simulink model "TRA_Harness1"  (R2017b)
settings: Solver=FixedStepDiscrete  StartTime=0.0  StopTime=16  FixedStep=0.01  RelTol=1e-3  EnableMultiTasking=on
undefined symbols (not defined in the file): sigbuilder_block
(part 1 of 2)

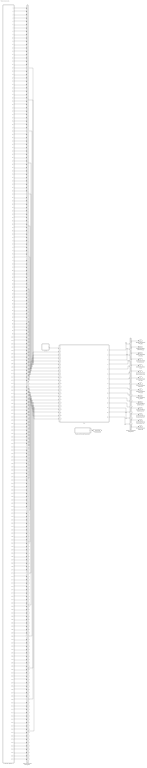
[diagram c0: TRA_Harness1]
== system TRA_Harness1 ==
  Chart : Stateflow chart  TreatAsAtomicUnit=on
  Harness Inputs : Subsystem  Tag=STV Subsys  LoadFcn=sigbuilder_block('load');  StartFcn=sigbuilder_block('start');  StopFcn=sigbuilder_block('stop');  ClipboardFcn=sigbuilder_block('clipboard');  mask(Sigbuilder block){tuvar=[0:10]}
      mask init:
      | if ~strcmp(get_param(bdroot(gcb),'SimulationStatus'),'stopped'),tuvar = sigbuilder_block('maskInit'); end
  Input Conversion Subsystem : Subsystem  Tag=__SLT_ICS__  Description=Signal spec. and routing
  Output Conversion Subsystem : Subsystem  Tag=__SLT_OCS__  Description=Signal spec. and routing
  Simulink Function scheduler : Test Sequence  Tag=__SLT_FCN_CALL__  TreatAsAtomicUnit=on
  TRA : ModelReference  ModelNameDialog=TRA  SimulationMode=Normal  ModelReferenceVersion='M112C123'
  GbTRA_ThmRnwyfDet_flg : Outport  OutDataTypeStr=boolean  PortDimensions=[1]
  GbTRA_TPLRnwyChkFinish_flg : Outport  Port=2  OutDataTypeStr=boolean  PortDimensions=[1]
  GbTRA_ShortSOCIDFit_flg : Outport  Port=3  OutDataTypeStr=boolean  PortDimensions=[1]
  GcTRA_ShortSOCMinID_numb : Outport  Port=4  OutDataTypeStr=uint8  PortDimensions=[1]
  GcTRA_RunTime_min : Outport  Port=5  OutDataTypeStr=uint16  PortDimensions=[1]
  GcTRA_ShortSOCRunTimeSum_min : Outport  Port=6  OutDataTypeStr=uint32  PortDimensions=[1]
  GcTRA_ShortSOCDiff_pct : Outport  Port=7  OutDataTypeStr=single  PortDimensions=[1]
  GbTRA_ThmRnwyWarn_flg : Outport  Port=8  OutDataTypeStr=boolean  PortDimensions=[1]
  GbTRA_ThmRnwyAlrm_flg : Outport  Port=9  OutDataTypeStr=boolean  PortDimensions=[1]
  GeTRA_ThmRnwySt_enum : Outport  Port=10  OutDataTypeStr=uint8  PortDimensions=[1]
  GcTRA_TPLWkupCellTemp_mV : Outport  Port=11  OutDataTypeStr=uint16  PortDimensions=[1]
  GcTRA_TPLWkupPCBTemp_mV : Outport  Port=12  OutDataTypeStr=uint16  PortDimensions=[1]
  GcTRA_TPLWkupCellVoltMax_mV : Outport  Port=13  OutDataTypeStr=uint16  PortDimensions=[1]
  GcTRA_TPLWkupCellVoltMin_mV : Outport  Port=14  OutDataTypeStr=uint16  PortDimensions=[1]
  GbTRA_TPLWkupEnable_flg : Outport  Port=15  OutDataTypeStr=boolean  PortDimensions=[1]
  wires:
  Harness Inputs/1(GcCDP_MaxCellTemp_C) -> Input Conversion Subsystem/1(Inport_1)
  Harness Inputs/2(GaCDP_CellTemp_C(1)) -> Input Conversion Subsystem/2(Inport_2)
  Harness Inputs/3(GaCDP_CellTemp_C(2)) -> Input Conversion Subsystem/3(Inport_3)
  Harness Inputs/4(GaCDP_CellTemp_C(3)) -> Input Conversion Subsystem/4(Inport_4)
  Harness Inputs/5(GaCDP_CellTemp_C(4)) -> Input Conversion Subsystem/5(Inport_5)
  Harness Inputs/6(GaCDP_CellTemp_C(5)) -> Input Conversion Subsystem/6(Inport_6)
  Harness Inputs/7(GaCDP_CellTemp_C(6)) -> Input Conversion Subsystem/7(Inport_7)
  Harness Inputs/8(GaCDP_CellTemp_C(7)) -> Input Conversion Subsystem/8(Inport_8)
  Harness Inputs/9(GaCDP_CellTemp_C(8)) -> Input Conversion Subsystem/9(Inport_9)
  Harness Inputs/10(GaCDP_CellTemp_C(9)) -> Input Conversion Subsystem/10(Inport_10)
  Harness Inputs/11(GaCDP_CellTemp_C(10)) -> Input Conversion Subsystem/11(Inport_11)
  Harness Inputs/12(GaCDP_CellTemp_C(11)) -> Input Conversion Subsystem/12(Inport_12)
  Harness Inputs/13(GaCDP_CellTemp_C(12)) -> Input Conversion Subsystem/13(Inport_13)
  Harness Inputs/14(GaCDP_CellTemp_C(13)) -> Input Conversion Subsystem/14(Inport_14)
  Harness Inputs/15(GaCDP_CellTemp_C(14)) -> Input Conversion Subsystem/15(Inport_15)
  Harness Inputs/16(GaCDP_CellTemp_C(15)) -> Input Conversion Subsystem/16(Inport_16)
  Harness Inputs/17(GaCDP_CellTemp_C(16)) -> Input Conversion Subsystem/17(Inport_17)
  Harness Inputs/18(GaCDP_CellTemp_C(17)) -> Input Conversion Subsystem/18(Inport_18)
  Harness Inputs/19(GaCDP_CellTemp_C(18)) -> Input Conversion Subsystem/19(Inport_19)
  Harness Inputs/20(GaCDP_CellTemp_C(19)) -> Input Conversion Subsystem/20(Inport_20)
  Harness Inputs/21(GaCDP_CellTemp_C(20)) -> Input Conversion Subsystem/21(Inport_21)
  Harness Inputs/22(GaCDP_CellTemp_C(21)) -> Input Conversion Subsystem/22(Inport_22)
  Harness Inputs/23(GaCDP_CellTemp_C(22)) -> Input Conversion Subsystem/23(Inport_23)
  Harness Inputs/24(GaCDP_CellTemp_C(23)) -> Input Conversion Subsystem/24(Inport_24)
  Harness Inputs/25(GaCDP_CellTemp_C(24)) -> Input Conversion Subsystem/25(Inport_25)
  Harness Inputs/26(GaCDP_CellTemp_C(25)) -> Input Conversion Subsystem/26(Inport_26)
  Harness Inputs/27(GaCDP_CellTemp_C(26)) -> Input Conversion Subsystem/27(Inport_27)
  Harness Inputs/28(GaCDP_CellTemp_C(27)) -> Input Conversion Subsystem/28(Inport_28)
  Harness Inputs/29(GaCDP_CellTemp_C(28)) -> Input Conversion Subsystem/29(Inport_29)
  Harness Inputs/30(GaCDP_CellTemp_C(29)) -> Input Conversion Subsystem/30(Inport_30)
  Harness Inputs/31(GaCDP_CellTemp_C(30)) -> Input Conversion Subsystem/31(Inport_31)
  Harness Inputs/32(GaCDP_CellTemp_C(31)) -> Input Conversion Subsystem/32(Inport_32)
  Harness Inputs/33(GaCDP_CellTemp_C(32)) -> Input Conversion Subsystem/33(Inport_33)
  Harness Inputs/34(GaCDP_CellTemp_C(33)) -> Input Conversion Subsystem/34(Inport_34)
  Harness Inputs/35(GaCDP_CellTemp_C(34)) -> Input Conversion Subsystem/35(Inport_35)
  Harness Inputs/36(GaCDP_CellTemp_C(35)) -> Input Conversion Subsystem/36(Inport_36)
  Harness Inputs/37(GaCDP_CellTemp_C(36)) -> Input Conversion Subsystem/37(Inport_37)
  Harness Inputs/38(GaCDP_CellTemp_C(37)) -> Input Conversion Subsystem/38(Inport_38)
  Harness Inputs/39(GaCDP_CellTemp_C(38)) -> Input Conversion Subsystem/39(Inport_39)
  Harness Inputs/40(GaCDP_CellTemp_C(39)) -> Input Conversion Subsystem/40(Inport_40)
  Harness Inputs/41(GaCDP_CellTemp_C(40)) -> Input Conversion Subsystem/41(Inport_41)
  Harness Inputs/42(GaCDP_CellTemp_C(41)) -> Input Conversion Subsystem/42(Inport_42)
  Harness Inputs/43(GaCDP_CellTemp_C(42)) -> Input Conversion Subsystem/43(Inport_43)
  Harness Inputs/44(GaCDP_CellTemp_C(43)) -> Input Conversion Subsystem/44(Inport_44)
  Harness Inputs/45(GaCDP_CellTemp_C(44)) -> Input Conversion Subsystem/45(Inport_45)
  Harness Inputs/46(GaCDP_CellTemp_C(45)) -> Input Conversion Subsystem/46(Inport_46)
  Harness Inputs/47(GaCDP_CellTemp_C(46)) -> Input Conversion Subsystem/47(Inport_47)
  Harness Inputs/48(GaCDP_CellTemp_C(47)) -> Input Conversion Subsystem/48(Inport_48)
  Harness Inputs/49(GaCDP_CellTemp_C(48)) -> Input Conversion Subsystem/49(Inport_49)
  Harness Inputs/50(GcCDP_MinCellTemp_C) -> Input Conversion Subsystem/50(Inport_50)
  Harness Inputs/51(GcUDS_CellTempNumb_numb) -> Input Conversion Subsystem/51(Inport_51)
  Harness Inputs/52(GcCDP_MaxBusbarTemp_C) -> Input Conversion Subsystem/52(Inport_52)
  Harness Inputs/53(GcCDP_MinBusbarTemp_C) -> Input Conversion Subsystem/53(Inport_53)
  Harness Inputs/54(GaCDP_BusbarTemp_C(1)) -> Input Conversion Subsystem/54(Inport_54)
  Harness Inputs/55(GaCDP_BusbarTemp_C(2)) -> Input Conversion Subsystem/55(Inport_55)
  Harness Inputs/56(GaCDP_BusbarTemp_C(3)) -> Input Conversion Subsystem/56(Inport_56)
  Harness Inputs/57(GaCDP_BusbarTemp_C(4)) -> Input Conversion Subsystem/57(Inport_57)
  Harness Inputs/58(GaCDP_BusbarTemp_C(5)) -> Input Conversion Subsystem/58(Inport_58)
  Harness Inputs/59(GaCDP_BusbarTemp_C(6)) -> Input Conversion Subsystem/59(Inport_59)
  Harness Inputs/60(GaCDP_BusbarTemp_C(7)) -> Input Conversion Subsystem/60(Inport_60)
  Harness Inputs/61(GaCDP_BusbarTemp_C(8)) -> Input Conversion Subsystem/61(Inport_61)
  Harness Inputs/62(GaCDP_BusbarTemp_C(9)) -> Input Conversion Subsystem/62(Inport_62)
  Harness Inputs/63(GaCDP_BusbarTemp_C(10)) -> Input Conversion Subsystem/63(Inport_63)
  Harness Inputs/64(GaCDP_BusbarTemp_C(11)) -> Input Conversion Subsystem/64(Inport_64)
  Harness Inputs/65(GaCDP_BusbarTemp_C(12)) -> Input Conversion Subsystem/65(Inport_65)
  Harness Inputs/66(GaCDP_BusbarTemp_C(13)) -> Input Conversion Subsystem/66(Inport_66)
  Harness Inputs/67(GaCDP_BusbarTemp_C(14)) -> Input Conversion Subsystem/67(Inport_67)
  Harness Inputs/68(GaCDP_BusbarTemp_C(15)) -> Input Conversion Subsystem/68(Inport_68)
  Harness Inputs/69(GaCDP_BusbarTemp_C(16)) -> Input Conversion Subsystem/69(Inport_69)
  Harness Inputs/70(GaCDP_BusbarTemp_C(17)) -> Input Conversion Subsystem/70(Inport_70)
  Harness Inputs/71(GaCDP_BusbarTemp_C(18)) -> Input Conversion Subsystem/71(Inport_71)
  Harness Inputs/72(GaCDP_BusbarTemp_C(19)) -> Input Conversion Subsystem/72(Inport_72)
  Harness Inputs/73(GaCDP_BusbarTemp_C(20)) -> Input Conversion Subsystem/73(Inport_73)
  Harness Inputs/74(GaCDP_BusbarTemp_C(21)) -> Input Conversion Subsystem/74(Inport_74)
  Harness Inputs/75(GaCDP_BusbarTemp_C(22)) -> Input Conversion Subsystem/75(Inport_75)
  Harness Inputs/76(GaCDP_BusbarTemp_C(23)) -> Input Conversion Subsystem/76(Inport_76)
  Harness Inputs/77(GaCDP_BusbarTemp_C(24)) -> Input Conversion Subsystem/77(Inport_77)
  Harness Inputs/78(GaCDP_BusbarTemp_C(25)) -> Input Conversion Subsystem/78(Inport_78)
  Harness Inputs/79(GaCDP_BusbarTemp_C(26)) -> Input Conversion Subsystem/79(Inport_79)
  Harness Inputs/80(GaCDP_BusbarTemp_C(27)) -> Input Conversion Subsystem/80(Inport_80)
  Harness Inputs/81(GaCDP_BusbarTemp_C(28)) -> Input Conversion Subsystem/81(Inport_81)
  Harness Inputs/82(GaCDP_BusbarTemp_C(29)) -> Input Conversion Subsystem/82(Inport_82)
  Harness Inputs/83(GaCDP_BusbarTemp_C(30)) -> Input Conversion Subsystem/83(Inport_83)
  Harness Inputs/84(GaCDP_BusbarTemp_C(31)) -> Input Conversion Subsystem/84(Inport_84)
  Harness Inputs/85(GaCDP_BusbarTemp_C(32)) -> Input Conversion Subsystem/85(Inport_85)
  Harness Inputs/86(GaCDP_BusbarTemp_C(33)) -> Input Conversion Subsystem/86(Inport_86)
  Harness Inputs/87(GaCDP_BusbarTemp_C(34)) -> Input Conversion Subsystem/87(Inport_87)
  Harness Inputs/88(GaCDP_BusbarTemp_C(35)) -> Input Conversion Subsystem/88(Inport_88)
  Harness Inputs/89(GaCDP_BusbarTemp_C(36)) -> Input Conversion Subsystem/89(Inport_89)
  Harness Inputs/90(GaCDP_BusbarTemp_C(37)) -> Input Conversion Subsystem/90(Inport_90)
  Harness Inputs/91(GaCDP_BusbarTemp_C(38)) -> Input Conversion Subsystem/91(Inport_91)
  Harness Inputs/92(GaCDP_BusbarTemp_C(39)) -> Input Conversion Subsystem/92(Inport_92)
  Harness Inputs/93(GaCDP_BusbarTemp_C(40)) -> Input Conversion Subsystem/93(Inport_93)
  Harness Inputs/94(GaCDP_BusbarTemp_C(41)) -> Input Conversion Subsystem/94(Inport_94)
  Harness Inputs/95(GaCDP_BusbarTemp_C(42)) -> Input Conversion Subsystem/95(Inport_95)
  Harness Inputs/96(GaCDP_BusbarTemp_C(43)) -> Input Conversion Subsystem/96(Inport_96)
  Harness Inputs/97(GaCDP_BusbarTemp_C(44)) -> Input Conversion Subsystem/97(Inport_97)
  Harness Inputs/98(GaCDP_BusbarTemp_C(45)) -> Input Conversion Subsystem/98(Inport_98)
  Harness Inputs/99(GaCDP_BusbarTemp_C(46)) -> Input Conversion Subsystem/99(Inport_99)
  Harness Inputs/100(GaCDP_BusbarTemp_C(47)) -> Input Conversion Subsystem/100(Inport_100)
  Harness Inputs/101(GaCDP_BusbarTemp_C(48)) -> Input Conversion Subsystem/101(Inport_101)
  Harness Inputs/102(GcUDS_BusbarTempNumb_numb) -> Input Conversion Subsystem/102(Inport_102)
  Harness Inputs/103(GeMSM_BMUState_enum) -> Input Conversion Subsystem/103(Inport_103)
  Harness Inputs/104(GbCDP_SumCellVoltVld_flg) -> Input Conversion Subsystem/104(Inport_104)
  Harness Inputs/105(GcRTC_SleepTime_min) -> Input Conversion Subsystem/105(Inport_105)
  Harness Inputs/106(GbNVM_ReadShortSOCIDFitVld_flg) -> Input Conversion Subsystem/106(Inport_106)
  Harness Inputs/107(GbNVM_ReadShortSOCMinIDVld_flg) -> Input Conversion Subsystem/107(Inport_107)
  Harness Inputs/108(GbNVM_ReadShortSOCDiffVld_flg) -> Input Conversion Subsystem/108(Inport_108)
  Harness Inputs/109(GbNVM_ReadShortSOCRunTiSumVld_flg) -> Input Conversion Subsystem/109(Inport_109)
  Harness Inputs/110(GaCDP_CellVolt_mV(1)) -> Input Conversion Subsystem/110(Inport_110)
  Harness Inputs/111(GaCDP_CellVolt_mV(2)) -> Input Conversion Subsystem/111(Inport_111)
  Harness Inputs/112(GaCDP_CellVolt_mV(3)) -> Input Conversion Subsystem/112(Inport_112)
  Harness Inputs/113(GaCDP_CellVolt_mV(4)) -> Input Conversion Subsystem/113(Inport_113)
  Harness Inputs/114(GaCDP_CellVolt_mV(5)) -> Input Conversion Subsystem/114(Inport_114)
  Harness Inputs/115(GaCDP_CellVolt_mV(6)) -> Input Conversion Subsystem/115(Inport_115)
  Harness Inputs/116(GaCDP_CellVolt_mV(7)) -> Input Conversion Subsystem/116(Inport_116)
  Harness Inputs/117(GaCDP_CellVolt_mV(8)) -> Input Conversion Subsystem/117(Inport_117)
  Harness Inputs/118(GaCDP_CellVolt_mV(9)) -> Input Conversion Subsystem/118(Inport_118)
  Harness Inputs/119(GaCDP_CellVolt_mV(10)) -> Input Conversion Subsystem/119(Inport_119)
  Harness Inputs/120(GaCDP_CellVolt_mV(11)) -> Input Conversion Subsystem/120(Inport_120)
  Harness Inputs/121(GaCDP_CellVolt_mV(12)) -> Input Conversion Subsystem/121(Inport_121)
  Harness Inputs/122(GaCDP_CellVolt_mV(13)) -> Input Conversion Subsystem/122(Inport_122)
  Harness Inputs/123(GaCDP_CellVolt_mV(14)) -> Input Conversion Subsystem/123(Inport_123)
  Harness Inputs/124(GaCDP_CellVolt_mV(15)) -> Input Conversion Subsystem/124(Inport_124)
  Harness Inputs/125(GaCDP_CellVolt_mV(16)) -> Input Conversion Subsystem/125(Inport_125)
  Harness Inputs/126(GaCDP_CellVolt_mV(17)) -> Input Conversion Subsystem/126(Inport_126)
  Harness Inputs/127(GaCDP_CellVolt_mV(18)) -> Input Conversion Subsystem/127(Inport_127)
  Harness Inputs/128(GaCDP_CellVolt_mV(19)) -> Input Conversion Subsystem/128(Inport_128)
  Harness Inputs/129(GaCDP_CellVolt_mV(20)) -> Input Conversion Subsystem/129(Inport_129)
  Harness Inputs/130(GaCDP_CellVolt_mV(21)) -> Input Conversion Subsystem/130(Inport_130)
  Harness Inputs/131(GaCDP_CellVolt_mV(22)) -> Input Conversion Subsystem/131(Inport_131)
  Harness Inputs/132(GaCDP_CellVolt_mV(23)) -> Input Conversion Subsystem/132(Inport_132)
  Harness Inputs/133(GaCDP_CellVolt_mV(24)) -> Input Conversion Subsystem/133(Inport_133)
  Harness Inputs/134(GaCDP_CellVolt_mV(25)) -> Input Conversion Subsystem/134(Inport_134)
  Harness Inputs/135(GaCDP_CellVolt_mV(26)) -> Input Conversion Subsystem/135(Inport_135)
  Harness Inputs/136(GaCDP_CellVolt_mV(27)) -> Input Conversion Subsystem/136(Inport_136)
  Harness Inputs/137(GaCDP_CellVolt_mV(28)) -> Input Conversion Subsystem/137(Inport_137)
  Harness Inputs/138(GaCDP_CellVolt_mV(29)) -> Input Conversion Subsystem/138(Inport_138)
  Harness Inputs/139(GaCDP_CellVolt_mV(30)) -> Input Conversion Subsystem/139(Inport_139)
  Harness Inputs/140(GaCDP_CellVolt_mV(31)) -> Input Conversion Subsystem/140(Inport_140)
  Harness Inputs/141(GaCDP_CellVolt_mV(32)) -> Input Conversion Subsystem/141(Inport_141)
  Harness Inputs/142(GaCDP_CellVolt_mV(33)) -> Input Conversion Subsystem/142(Inport_142)
  Harness Inputs/143(GaCDP_CellVolt_mV(34)) -> Input Conversion Subsystem/143(Inport_143)
  Harness Inputs/144(GaCDP_CellVolt_mV(35)) -> Input Conversion Subsystem/144(Inport_144)
  Harness Inputs/145(GaCDP_CellVolt_mV(36)) -> Input Conversion Subsystem/145(Inport_145)
  Harness Inputs/146(GaCDP_CellVolt_mV(37)) -> Input Conversion Subsystem/146(Inport_146)
  Harness Inputs/147(GaCDP_CellVolt_mV(38)) -> Input Conversion Subsystem/147(Inport_147)
  Harness Inputs/148(GaCDP_CellVolt_mV(39)) -> Input Conversion Subsystem/148(Inport_148)
  Harness Inputs/149(GaCDP_CellVolt_mV(40)) -> Input Conversion Subsystem/149(Inport_149)
  Harness Inputs/150(GaCDP_CellVolt_mV(41)) -> Input Conversion Subsystem/150(Inport_150)
  Harness Inputs/151(GaCDP_CellVolt_mV(42)) -> Input Conversion Subsystem/151(Inport_151)
  Harness Inputs/152(GaCDP_CellVolt_mV(43)) -> Input Conversion Subsystem/152(Inport_152)
  Harness Inputs/153(GaCDP_CellVolt_mV(44)) -> Input Conversion Subsystem/153(Inport_153)
  Harness Inputs/154(GaCDP_CellVolt_mV(45)) -> Input Conversion Subsystem/154(Inport_154)
  Harness Inputs/155(GaCDP_CellVolt_mV(46)) -> Input Conversion Subsystem/155(Inport_155)
  Harness Inputs/156(GaCDP_CellVolt_mV(47)) -> Input Conversion Subsystem/156(Inport_156)
  Harness Inputs/157(GaCDP_CellVolt_mV(48)) -> Input Conversion Subsystem/157(Inport_157)
  Harness Inputs/158(GaCDP_CellVolt_mV(49)) -> Input Conversion Subsystem/158(Inport_158)
  Harness Inputs/159(GaCDP_CellVolt_mV(50)) -> Input Conversion Subsystem/159(Inport_159)
  Harness Inputs/160(GaCDP_CellVolt_mV(51)) -> Input Conversion Subsystem/160(Inport_160)
  Harness Inputs/161(GaCDP_CellVolt_mV(52)) -> Input Conversion Subsystem/161(Inport_161)
  Harness Inputs/162(GaCDP_CellVolt_mV(53)) -> Input Conversion Subsystem/162(Inport_162)
  Harness Inputs/163(GaCDP_CellVolt_mV(54)) -> Input Conversion Subsystem/163(Inport_163)
  Harness Inputs/164(GaCDP_CellVolt_mV(55)) -> Input Conversion Subsystem/164(Inport_164)
  Harness Inputs/165(GaCDP_CellVolt_mV(56)) -> Input Conversion Subsystem/165(Inport_165)
  Harness Inputs/166(GaCDP_CellVolt_mV(57)) -> Input Conversion Subsystem/166(Inport_166)
  Harness Inputs/167(GaCDP_CellVolt_mV(58)) -> Input Conversion Subsystem/167(Inport_167)
  Harness Inputs/168(GaCDP_CellVolt_mV(59)) -> Input Conversion Subsystem/168(Inport_168)
  Harness Inputs/169(GaCDP_CellVolt_mV(60)) -> Input Conversion Subsystem/169(Inport_169)
  Harness Inputs/170(GaCDP_CellVolt_mV(61)) -> Input Conversion Subsystem/170(Inport_170)
  Harness Inputs/171(GaCDP_CellVolt_mV(62)) -> Input Conversion Subsystem/171(Inport_171)
  Harness Inputs/172(GaCDP_CellVolt_mV(63)) -> Input Conversion Subsystem/172(Inport_172)
  Harness Inputs/173(GaCDP_CellVolt_mV(64)) -> Input Conversion Subsystem/173(Inport_173)
  Harness Inputs/174(GaCDP_CellVolt_mV(65)) -> Input Conversion Subsystem/174(Inport_174)
  Harness Inputs/175(GaCDP_CellVolt_mV(66)) -> Input Conversion Subsystem/175(Inport_175)
  Harness Inputs/176(GaCDP_CellVolt_mV(67)) -> Input Conversion Subsystem/176(Inport_176)
  Harness Inputs/177(GaCDP_CellVolt_mV(68)) -> Input Conversion Subsystem/177(Inport_177)
  Harness Inputs/178(GaCDP_CellVolt_mV(69)) -> Input Conversion Subsystem/178(Inport_178)
  Harness Inputs/179(GaCDP_CellVolt_mV(70)) -> Input Conversion Subsystem/179(Inport_179)
  Harness Inputs/180(GaCDP_CellVolt_mV(71)) -> Input Conversion Subsystem/180(Inport_180)
  Harness Inputs/181(GaCDP_CellVolt_mV(72)) -> Input Conversion Subsystem/181(Inport_181)
  Harness Inputs/182(GaCDP_CellVolt_mV(73)) -> Input Conversion Subsystem/182(Inport_182)
  Harness Inputs/183(GaCDP_CellVolt_mV(74)) -> Input Conversion Subsystem/183(Inport_183)
  Harness Inputs/184(GaCDP_CellVolt_mV(75)) -> Input Conversion Subsystem/184(Inport_184)
  Harness Inputs/185(GaCDP_CellVolt_mV(76)) -> Input Conversion Subsystem/185(Inport_185)
  Harness Inputs/186(GaCDP_CellVolt_mV(77)) -> Input Conversion Subsystem/186(Inport_186)
  Harness Inputs/187(GaCDP_CellVolt_mV(78)) -> Input Conversion Subsystem/187(Inport_187)
  Harness Inputs/188(GaCDP_CellVolt_mV(79)) -> Input Conversion Subsystem/188(Inport_188)
  Harness Inputs/189(GaCDP_CellVolt_mV(80)) -> Input Conversion Subsystem/189(Inport_189)
  Harness Inputs/190(GaCDP_CellVolt_mV(81)) -> Input Conversion Subsystem/190(Inport_190)
  Harness Inputs/191(GaCDP_CellVolt_mV(82)) -> Input Conversion Subsystem/191(Inport_191)
  Harness Inputs/192(GaCDP_CellVolt_mV(83)) -> Input Conversion Subsystem/192(Inport_192)
  Harness Inputs/193(GaCDP_CellVolt_mV(84)) -> Input Conversion Subsystem/193(Inport_193)
  Harness Inputs/194(GaCDP_CellVolt_mV(85)) -> Input Conversion Subsystem/194(Inport_194)
  Harness Inputs/195(GaCDP_CellVolt_mV(86)) -> Input Conversion Subsystem/195(Inport_195)
  Harness Inputs/196(GaCDP_CellVolt_mV(87)) -> Input Conversion Subsystem/196(Inport_196)
  Harness Inputs/197(GaCDP_CellVolt_mV(88)) -> Input Conversion Subsystem/197(Inport_197)
  Harness Inputs/198(GaCDP_CellVolt_mV(89)) -> Input Conversion Subsystem/198(Inport_198)
  Harness Inputs/199(GaCDP_CellVolt_mV(90)) -> Input Conversion Subsystem/199(Inport_199)
  Harness Inputs/200(GaCDP_CellVolt_mV(91)) -> Input Conversion Subsystem/200(Inport_200)
  Harness Inputs/201(GaCDP_CellVolt_mV(92)) -> Input Conversion Subsystem/201(Inport_201)
  Harness Inputs/202(GaCDP_CellVolt_mV(93)) -> Input Conversion Subsystem/202(Inport_202)
  Harness Inputs/203(GaCDP_CellVolt_mV(94)) -> Input Conversion Subsystem/203(Inport_203)
  Harness Inputs/204(GaCDP_CellVolt_mV(95)) -> Input Conversion Subsystem/204(Inport_204)
  Harness Inputs/205(GaCDP_CellVolt_mV(96)) -> Input Conversion Subsystem/205(Inport_205)
  Harness Inputs/206(GaCDP_CellVolt_mV(97)) -> Input Conversion Subsystem/206(Inport_206)
  Harness Inputs/207(GaCDP_CellVolt_mV(98)) -> Input Conversion Subsystem/207(Inport_207)
  Harness Inputs/208(GaCDP_CellVolt_mV(99)) -> Input Conversion Subsystem/208(Inport_208)
  Harness Inputs/209(GaCDP_CellVolt_mV(100)) -> Input Conversion Subsystem/209(Inport_209)
  Harness Inputs/210(GaCDP_CellVolt_mV(101)) -> Input Conversion Subsystem/210(Inport_210)
  Harness Inputs/211(GaCDP_CellVolt_mV(102)) -> Input Conversion Subsystem/211(Inport_211)
  Harness Inputs/212(GaCDP_CellVolt_mV(103)) -> Input Conversion Subsystem/212(Inport_212)
  Harness Inputs/213(GaCDP_CellVolt_mV(104)) -> Input Conversion Subsystem/213(Inport_213)
  Harness Inputs/214(GaCDP_CellVolt_mV(105)) -> Input Conversion Subsystem/214(Inport_214)
  Harness Inputs/215(GaCDP_CellVolt_mV(106)) -> Input Conversion Subsystem/215(Inport_215)
  Harness Inputs/216(GaCDP_CellVolt_mV(107)) -> Input Conversion Subsystem/216(Inport_216)
  Harness Inputs/217(GaCDP_CellVolt_mV(108)) -> Input Conversion Subsystem/217(Inport_217)
  Harness Inputs/218(GaCDP_CellVolt_mV(109)) -> Input Conversion Subsystem/218(Inport_218)
  Harness Inputs/219(GaCDP_CellVolt_mV(110)) -> Input Conversion Subsystem/219(Inport_219)
  Harness Inputs/220(GaCDP_CellVolt_mV(111)) -> Input Conversion Subsystem/220(Inport_220)
  Harness Inputs/221(GaCDP_CellVolt_mV(112)) -> Input Conversion Subsystem/221(Inport_221)
  Harness Inputs/222(GeUDS_CapSel_enum) -> Input Conversion Subsystem/222(Inport_222)
  Harness Inputs/223(GbNVM_ReadLastShortSOCRunTiVld_flg) -> Input Conversion Subsystem/223(Inport_223)
  Harness Inputs/224(GcCDP_AvgCellVolt_mV) -> Input Conversion Subsystem/224(Inport_224)
  Harness Inputs/225(GcUDS_CellVoltNum_numb) -> Input Conversion Subsystem/225(Inport_225)
  Harness Inputs/226(GcHDP_PackCrnt_A) -> Input Conversion Subsystem/226(Inport_226)
  Harness Inputs/227(GeISP_WkUpSrcSt_enum) -> Input Conversion Subsystem/227(Inport_227)
  Output Conversion Subsystem/1(Outport_1) -> GbTRA_ThmRnwyfDet_flg/1
  Output Conversion Subsystem/2(Outport_2) -> GbTRA_TPLRnwyChkFinish_flg/1
  Output Conversion Subsystem/3(Outport_3) -> GbTRA_ShortSOCIDFit_flg/1
  Output Conversion Subsystem/4(Outport_4) -> GcTRA_ShortSOCMinID_numb/1
  Output Conversion Subsystem/5(Outport_5) -> GcTRA_RunTime_min/1
  Output Conversion Subsystem/6(Outport_6) -> GcTRA_ShortSOCRunTimeSum_min/1
  Output Conversion Subsystem/7(Outport_7) -> GcTRA_ShortSOCDiff_pct/1
  Output Conversion Subsystem/8(Outport_8) -> GbTRA_ThmRnwyWarn_flg/1
  Output Conversion Subsystem/9(Outport_9) -> GbTRA_ThmRnwyAlrm_flg/1
  Output Conversion Subsystem/10(Outport_10) -> GeTRA_ThmRnwySt_enum/1
  Output Conversion Subsystem/11(Outport_11) -> GcTRA_TPLWkupCellTemp_mV/1
  Output Conversion Subsystem/12(Outport_12) -> GcTRA_TPLWkupPCBTemp_mV/1
  Output Conversion Subsystem/13(Outport_13) -> GcTRA_TPLWkupCellVoltMax_mV/1
  Output Conversion Subsystem/14(Outport_14) -> GcTRA_TPLWkupCellVoltMin_mV/1
  Output Conversion Subsystem/15(Outport_15) -> GbTRA_TPLWkupEnable_flg/1
  Input Conversion Subsystem/2(Outport_2) -> TRA/2
  Input Conversion Subsystem/3(Outport_3) -> TRA/3
  Input Conversion Subsystem/4(Outport_4) -> TRA/4
  Input Conversion Subsystem/5(Outport_5) -> TRA/5
  Input Conversion Subsystem/6(Outport_6) -> TRA/6
  Input Conversion Subsystem/7(Outport_7) -> TRA/7
  Input Conversion Subsystem/8(Outport_8) -> TRA/8
  Input Conversion Subsystem/9(Outport_9) -> TRA/9
  Input Conversion Subsystem/10(Outport_10) -> TRA/10
  Input Conversion Subsystem/11(Outport_11) -> TRA/11
  Input Conversion Subsystem/12(Outport_12) -> TRA/12
  Input Conversion Subsystem/13(Outport_13) -> TRA/13
  Input Conversion Subsystem/14(Outport_14) -> TRA/14
  Input Conversion Subsystem/15(Outport_15) -> TRA/15
  Input Conversion Subsystem/16(Outport_16) -> TRA/16
  Input Conversion Subsystem/17(Outport_17) -> TRA/17
  Input Conversion Subsystem/18(Outport_18) -> TRA/18
  Input Conversion Subsystem/19(Outport_19) -> TRA/19
  Input Conversion Subsystem/20(Outport_20) -> TRA/20
  Input Conversion Subsystem/21(Outport_21) -> TRA/21
  Input Conversion Subsystem/22(Outport_22) -> TRA/22
  Input Conversion Subsystem/23(Outport_23) -> TRA/23
  TRA/1 -> Output Conversion Subsystem/1(Inport_1)
  TRA/2 -> Output Conversion Subsystem/2(Inport_2)
  TRA/3 -> Output Conversion Subsystem/3(Inport_3)
  TRA/4 -> Output Conversion Subsystem/4(Inport_4)
  TRA/5 -> Output Conversion Subsystem/5(Inport_5)
  TRA/6 -> Output Conversion Subsystem/6(Inport_6)
  TRA/7 -> Output Conversion Subsystem/7(Inport_7)
  TRA/8 -> Output Conversion Subsystem/8(Inport_8)
  TRA/9 -> Output Conversion Subsystem/9(Inport_9)
  TRA/10 -> Output Conversion Subsystem/10(Inport_10)
  TRA/11 -> Output Conversion Subsystem/11(Inport_11)
  TRA/12 -> Output Conversion Subsystem/12(Inport_12)
  TRA/13 -> Output Conversion Subsystem/13(Inport_13)
  TRA/14 -> Output Conversion Subsystem/14(Inport_14)
  TRA/15 -> Output Conversion Subsystem/15(Inport_15)
  Simulink Function scheduler/1(TRA_ThemRunAway_10ms()) -> [send_fcn1]
  Chart/1(Run10ms()) -> TRA/1

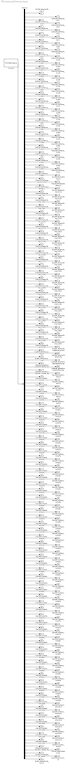
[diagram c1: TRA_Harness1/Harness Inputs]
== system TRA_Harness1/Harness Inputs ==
  Demux : Demux  Tag=STV Demux  Outputs=227
  FromWs : FromWorkspace  Tag=STV FromWs  VariableName=tuvar  SampleTime=0
  GcCDP_MaxCellTemp_C : Outport  Tag=STV Outport
  GaCDP_CellTemp_C(1) : Outport  Tag=STV Outport  Port=2
  GaCDP_CellTemp_C(2) : Outport  Tag=STV Outport  Port=3
  GaCDP_CellTemp_C(3) : Outport  Tag=STV Outport  Port=4
  GaCDP_CellTemp_C(4) : Outport  Tag=STV Outport  Port=5
  GaCDP_CellTemp_C(5) : Outport  Tag=STV Outport  Port=6
  GaCDP_CellTemp_C(6) : Outport  Tag=STV Outport  Port=7
  GaCDP_CellTemp_C(7) : Outport  Tag=STV Outport  Port=8
  GaCDP_CellTemp_C(8) : Outport  Tag=STV Outport  Port=9
  GaCDP_CellTemp_C(9) : Outport  Tag=STV Outport  Port=10
  GaCDP_CellTemp_C(10) : Outport  Tag=STV Outport  Port=11
  GaCDP_CellTemp_C(11) : Outport  Tag=STV Outport  Port=12
  GaCDP_CellTemp_C(12) : Outport  Tag=STV Outport  Port=13
  GaCDP_CellTemp_C(13) : Outport  Tag=STV Outport  Port=14
  GaCDP_CellTemp_C(14) : Outport  Tag=STV Outport  Port=15
  GaCDP_CellTemp_C(15) : Outport  Tag=STV Outport  Port=16
  GaCDP_CellTemp_C(16) : Outport  Tag=STV Outport  Port=17
  GaCDP_CellTemp_C(17) : Outport  Tag=STV Outport  Port=18
  GaCDP_CellTemp_C(18) : Outport  Tag=STV Outport  Port=19
  GaCDP_CellTemp_C(19) : Outport  Tag=STV Outport  Port=20
  GaCDP_CellTemp_C(20) : Outport  Tag=STV Outport  Port=21
  GaCDP_CellTemp_C(21) : Outport  Tag=STV Outport  Port=22
  GaCDP_CellTemp_C(22) : Outport  Tag=STV Outport  Port=23
  GaCDP_CellTemp_C(23) : Outport  Tag=STV Outport  Port=24
  GaCDP_CellTemp_C(24) : Outport  Tag=STV Outport  Port=25
  GaCDP_CellTemp_C(25) : Outport  Tag=STV Outport  Port=26
  GaCDP_CellTemp_C(26) : Outport  Tag=STV Outport  Port=27
  GaCDP_CellTemp_C(27) : Outport  Tag=STV Outport  Port=28
  GaCDP_CellTemp_C(28) : Outport  Tag=STV Outport  Port=29
  GaCDP_CellTemp_C(29) : Outport  Tag=STV Outport  Port=30
  GaCDP_CellTemp_C(30) : Outport  Tag=STV Outport  Port=31
  GaCDP_CellTemp_C(31) : Outport  Tag=STV Outport  Port=32
  GaCDP_CellTemp_C(32) : Outport  Tag=STV Outport  Port=33
  GaCDP_CellTemp_C(33) : Outport  Tag=STV Outport  Port=34
  GaCDP_CellTemp_C(34) : Outport  Tag=STV Outport  Port=35
  GaCDP_CellTemp_C(35) : Outport  Tag=STV Outport  Port=36
  GaCDP_CellTemp_C(36) : Outport  Tag=STV Outport  Port=37
  GaCDP_CellTemp_C(37) : Outport  Tag=STV Outport  Port=38
  GaCDP_CellTemp_C(38) : Outport  Tag=STV Outport  Port=39
  GaCDP_CellTemp_C(39) : Outport  Tag=STV Outport  Port=40
  GaCDP_CellTemp_C(40) : Outport  Tag=STV Outport  Port=41
  GaCDP_CellTemp_C(41) : Outport  Tag=STV Outport  Port=42
  GaCDP_CellTemp_C(42) : Outport  Tag=STV Outport  Port=43
  GaCDP_CellTemp_C(43) : Outport  Tag=STV Outport  Port=44
  GaCDP_CellTemp_C(44) : Outport  Tag=STV Outport  Port=45
  GaCDP_CellTemp_C(45) : Outport  Tag=STV Outport  Port=46
  GaCDP_CellTemp_C(46) : Outport  Tag=STV Outport  Port=47
  GaCDP_CellTemp_C(47) : Outport  Tag=STV Outport  Port=48
  GaCDP_CellTemp_C(48) : Outport  Tag=STV Outport  Port=49
  GcCDP_MinCellTemp_C : Outport  Tag=STV Outport  Port=50
  GcUDS_CellTempNumb_numb : Outport  Tag=STV Outport  Port=51
  GcCDP_MaxBusbarTemp_C : Outport  Tag=STV Outport  Port=52
  GcCDP_MinBusbarTemp_C : Outport  Tag=STV Outport  Port=53
  GaCDP_BusbarTemp_C(1) : Outport  Tag=STV Outport  Port=54
  GaCDP_BusbarTemp_C(2) : Outport  Tag=STV Outport  Port=55
  GaCDP_BusbarTemp_C(3) : Outport  Tag=STV Outport  Port=56
  GaCDP_BusbarTemp_C(4) : Outport  Tag=STV Outport  Port=57
  GaCDP_BusbarTemp_C(5) : Outport  Tag=STV Outport  Port=58
  GaCDP_BusbarTemp_C(6) : Outport  Tag=STV Outport  Port=59
  GaCDP_BusbarTemp_C(7) : Outport  Tag=STV Outport  Port=60
  GaCDP_BusbarTemp_C(8) : Outport  Tag=STV Outport  Port=61
  GaCDP_BusbarTemp_C(9) : Outport  Tag=STV Outport  Port=62
  GaCDP_BusbarTemp_C(10) : Outport  Tag=STV Outport  Port=63
  GaCDP_BusbarTemp_C(11) : Outport  Tag=STV Outport  Port=64
  GaCDP_BusbarTemp_C(12) : Outport  Tag=STV Outport  Port=65
  GaCDP_BusbarTemp_C(13) : Outport  Tag=STV Outport  Port=66
  GaCDP_BusbarTemp_C(14) : Outport  Tag=STV Outport  Port=67
  GaCDP_BusbarTemp_C(15) : Outport  Tag=STV Outport  Port=68
  GaCDP_BusbarTemp_C(16) : Outport  Tag=STV Outport  Port=69
  GaCDP_BusbarTemp_C(17) : Outport  Tag=STV Outport  Port=70
  GaCDP_BusbarTemp_C(18) : Outport  Tag=STV Outport  Port=71
  GaCDP_BusbarTemp_C(19) : Outport  Tag=STV Outport  Port=72
  GaCDP_BusbarTemp_C(20) : Outport  Tag=STV Outport  Port=73
  GaCDP_BusbarTemp_C(21) : Outport  Tag=STV Outport  Port=74
  GaCDP_BusbarTemp_C(22) : Outport  Tag=STV Outport  Port=75
  GaCDP_BusbarTemp_C(23) : Outport  Tag=STV Outport  Port=76
  GaCDP_BusbarTemp_C(24) : Outport  Tag=STV Outport  Port=77
  GaCDP_BusbarTemp_C(25) : Outport  Tag=STV Outport  Port=78
  GaCDP_BusbarTemp_C(26) : Outport  Tag=STV Outport  Port=79
  GaCDP_BusbarTemp_C(27) : Outport  Tag=STV Outport  Port=80
  GaCDP_BusbarTemp_C(28) : Outport  Tag=STV Outport  Port=81
  GaCDP_BusbarTemp_C(29) : Outport  Tag=STV Outport  Port=82
  GaCDP_BusbarTemp_C(30) : Outport  Tag=STV Outport  Port=83
  GaCDP_BusbarTemp_C(31) : Outport  Tag=STV Outport  Port=84
  GaCDP_BusbarTemp_C(32) : Outport  Tag=STV Outport  Port=85
  GaCDP_BusbarTemp_C(33) : Outport  Tag=STV Outport  Port=86
  GaCDP_BusbarTemp_C(34) : Outport  Tag=STV Outport  Port=87
  GaCDP_BusbarTemp_C(35) : Outport  Tag=STV Outport  Port=88
  GaCDP_BusbarTemp_C(36) : Outport  Tag=STV Outport  Port=89
  GaCDP_BusbarTemp_C(37) : Outport  Tag=STV Outport  Port=90
  GaCDP_BusbarTemp_C(38) : Outport  Tag=STV Outport  Port=91
  GaCDP_BusbarTemp_C(39) : Outport  Tag=STV Outport  Port=92
  GaCDP_BusbarTemp_C(40) : Outport  Tag=STV Outport  Port=93
  GaCDP_BusbarTemp_C(41) : Outport  Tag=STV Outport  Port=94
  GaCDP_BusbarTemp_C(42) : Outport  Tag=STV Outport  Port=95
  GaCDP_BusbarTemp_C(43) : Outport  Tag=STV Outport  Port=96
  GaCDP_BusbarTemp_C(44) : Outport  Tag=STV Outport  Port=97
  GaCDP_BusbarTemp_C(45) : Outport  Tag=STV Outport  Port=98
  GaCDP_BusbarTemp_C(46) : Outport  Tag=STV Outport  Port=99
  GaCDP_BusbarTemp_C(47) : Outport  Tag=STV Outport  Port=100
  GaCDP_BusbarTemp_C(48) : Outport  Tag=STV Outport  Port=101
  GcUDS_BusbarTempNumb_numb : Outport  Tag=STV Outport  Port=102
  GeMSM_BMUState_enum : Outport  Tag=STV Outport  Port=103
  GbCDP_SumCellVoltVld_flg : Outport  Tag=STV Outport  Port=104
  GcRTC_SleepTime_min : Outport  Tag=STV Outport  Port=105
  GbNVM_ReadShortSOCIDFitVld_flg : Outport  Tag=STV Outport  Port=106
  GbNVM_ReadShortSOCMinIDVld_flg : Outport  Tag=STV Outport  Port=107
  GbNVM_ReadShortSOCDiffVld_flg : Outport  Tag=STV Outport  Port=108
  GbNVM_ReadShortSOCRunTiSumVld_flg : Outport  Tag=STV Outport  Port=109
  GaCDP_CellVolt_mV(1) : Outport  Tag=STV Outport  Port=110
  GaCDP_CellVolt_mV(2) : Outport  Tag=STV Outport  Port=111
  GaCDP_CellVolt_mV(3) : Outport  Tag=STV Outport  Port=112
  GaCDP_CellVolt_mV(4) : Outport  Tag=STV Outport  Port=113
  GaCDP_CellVolt_mV(5) : Outport  Tag=STV Outport  Port=114
  GaCDP_CellVolt_mV(6) : Outport  Tag=STV Outport  Port=115
  GaCDP_CellVolt_mV(7) : Outport  Tag=STV Outport  Port=116
  GaCDP_CellVolt_mV(8) : Outport  Tag=STV Outport  Port=117
  GaCDP_CellVolt_mV(9) : Outport  Tag=STV Outport  Port=118
  GaCDP_CellVolt_mV(10) : Outport  Tag=STV Outport  Port=119
  GaCDP_CellVolt_mV(11) : Outport  Tag=STV Outport  Port=120
  GaCDP_CellVolt_mV(12) : Outport  Tag=STV Outport  Port=121
  GaCDP_CellVolt_mV(13) : Outport  Tag=STV Outport  Port=122
  GaCDP_CellVolt_mV(14) : Outport  Tag=STV Outport  Port=123
  GaCDP_CellVolt_mV(15) : Outport  Tag=STV Outport  Port=124
  GaCDP_CellVolt_mV(16) : Outport  Tag=STV Outport  Port=125
  GaCDP_CellVolt_mV(17) : Outport  Tag=STV Outport  Port=126
  GaCDP_CellVolt_mV(18) : Outport  Tag=STV Outport  Port=127
  GaCDP_CellVolt_mV(19) : Outport  Tag=STV Outport  Port=128
  GaCDP_CellVolt_mV(20) : Outport  Tag=STV Outport  Port=129
  GaCDP_CellVolt_mV(21) : Outport  Tag=STV Outport  Port=130
  GaCDP_CellVolt_mV(22) : Outport  Tag=STV Outport  Port=131
  GaCDP_CellVolt_mV(23) : Outport  Tag=STV Outport  Port=132
  GaCDP_CellVolt_mV(24) : Outport  Tag=STV Outport  Port=133
  GaCDP_CellVolt_mV(25) : Outport  Tag=STV Outport  Port=134
  GaCDP_CellVolt_mV(26) : Outport  Tag=STV Outport  Port=135
  GaCDP_CellVolt_mV(27) : Outport  Tag=STV Outport  Port=136
  GaCDP_CellVolt_mV(28) : Outport  Tag=STV Outport  Port=137
  GaCDP_CellVolt_mV(29) : Outport  Tag=STV Outport  Port=138
  GaCDP_CellVolt_mV(30) : Outport  Tag=STV Outport  Port=139
  GaCDP_CellVolt_mV(31) : Outport  Tag=STV Outport  Port=140
  GaCDP_CellVolt_mV(32) : Outport  Tag=STV Outport  Port=141
  GaCDP_CellVolt_mV(33) : Outport  Tag=STV Outport  Port=142
  GaCDP_CellVolt_mV(34) : Outport  Tag=STV Outport  Port=143
  GaCDP_CellVolt_mV(35) : Outport  Tag=STV Outport  Port=144
  GaCDP_CellVolt_mV(36) : Outport  Tag=STV Outport  Port=145
  GaCDP_CellVolt_mV(37) : Outport  Tag=STV Outport  Port=146
  GaCDP_CellVolt_mV(38) : Outport  Tag=STV Outport  Port=147
  GaCDP_CellVolt_mV(39) : Outport  Tag=STV Outport  Port=148
  GaCDP_CellVolt_mV(40) : Outport  Tag=STV Outport  Port=149
  GaCDP_CellVolt_mV(41) : Outport  Tag=STV Outport  Port=150
  GaCDP_CellVolt_mV(42) : Outport  Tag=STV Outport  Port=151
  GaCDP_CellVolt_mV(43) : Outport  Tag=STV Outport  Port=152
  GaCDP_CellVolt_mV(44) : Outport  Tag=STV Outport  Port=153
  GaCDP_CellVolt_mV(45) : Outport  Tag=STV Outport  Port=154
  GaCDP_CellVolt_mV(46) : Outport  Tag=STV Outport  Port=155
  GaCDP_CellVolt_mV(47) : Outport  Tag=STV Outport  Port=156
  GaCDP_CellVolt_mV(48) : Outport  Tag=STV Outport  Port=157
  GaCDP_CellVolt_mV(49) : Outport  Tag=STV Outport  Port=158
  GaCDP_CellVolt_mV(50) : Outport  Tag=STV Outport  Port=159
  GaCDP_CellVolt_mV(51) : Outport  Tag=STV Outport  Port=160
  GaCDP_CellVolt_mV(52) : Outport  Tag=STV Outport  Port=161
  GaCDP_CellVolt_mV(53) : Outport  Tag=STV Outport  Port=162
  GaCDP_CellVolt_mV(54) : Outport  Tag=STV Outport  Port=163
  GaCDP_CellVolt_mV(55) : Outport  Tag=STV Outport  Port=164
  GaCDP_CellVolt_mV(56) : Outport  Tag=STV Outport  Port=165
  GaCDP_CellVolt_mV(57) : Outport  Tag=STV Outport  Port=166
  GaCDP_CellVolt_mV(58) : Outport  Tag=STV Outport  Port=167
  GaCDP_CellVolt_mV(59) : Outport  Tag=STV Outport  Port=168
  GaCDP_CellVolt_mV(60) : Outport  Tag=STV Outport  Port=169
  GaCDP_CellVolt_mV(61) : Outport  Tag=STV Outport  Port=170
  GaCDP_CellVolt_mV(62) : Outport  Tag=STV Outport  Port=171
  GaCDP_CellVolt_mV(63) : Outport  Tag=STV Outport  Port=172
  GaCDP_CellVolt_mV(64) : Outport  Tag=STV Outport  Port=173
  GaCDP_CellVolt_mV(65) : Outport  Tag=STV Outport  Port=174
  GaCDP_CellVolt_mV(66) : Outport  Tag=STV Outport  Port=175
  GaCDP_CellVolt_mV(67) : Outport  Tag=STV Outport  Port=176
  GaCDP_CellVolt_mV(68) : Outport  Tag=STV Outport  Port=177
  GaCDP_CellVolt_mV(69) : Outport  Tag=STV Outport  Port=178
  GaCDP_CellVolt_mV(70) : Outport  Tag=STV Outport  Port=179
  GaCDP_CellVolt_mV(71) : Outport  Tag=STV Outport  Port=180
  GaCDP_CellVolt_mV(72) : Outport  Tag=STV Outport  Port=181
  GaCDP_CellVolt_mV(73) : Outport  Tag=STV Outport  Port=182
  GaCDP_CellVolt_mV(74) : Outport  Tag=STV Outport  Port=183
  GaCDP_CellVolt_mV(75) : Outport  Tag=STV Outport  Port=184
  GaCDP_CellVolt_mV(76) : Outport  Tag=STV Outport  Port=185
  GaCDP_CellVolt_mV(77) : Outport  Tag=STV Outport  Port=186
  GaCDP_CellVolt_mV(78) : Outport  Tag=STV Outport  Port=187
  GaCDP_CellVolt_mV(79) : Outport  Tag=STV Outport  Port=188
  GaCDP_CellVolt_mV(80) : Outport  Tag=STV Outport  Port=189
  GaCDP_CellVolt_mV(81) : Outport  Tag=STV Outport  Port=190
  GaCDP_CellVolt_mV(82) : Outport  Tag=STV Outport  Port=191
  GaCDP_CellVolt_mV(83) : Outport  Tag=STV Outport  Port=192
  GaCDP_CellVolt_mV(84) : Outport  Tag=STV Outport  Port=193
  GaCDP_CellVolt_mV(85) : Outport  Tag=STV Outport  Port=194
  GaCDP_CellVolt_mV(86) : Outport  Tag=STV Outport  Port=195
  GaCDP_CellVolt_mV(87) : Outport  Tag=STV Outport  Port=196
  GaCDP_CellVolt_mV(88) : Outport  Tag=STV Outport  Port=197
  GaCDP_CellVolt_mV(89) : Outport  Tag=STV Outport  Port=198
  GaCDP_CellVolt_mV(90) : Outport  Tag=STV Outport  Port=199
  GaCDP_CellVolt_mV(91) : Outport  Tag=STV Outport  Port=200
  GaCDP_CellVolt_mV(92) : Outport  Tag=STV Outport  Port=201
  GaCDP_CellVolt_mV(93) : Outport  Tag=STV Outport  Port=202
  GaCDP_CellVolt_mV(94) : Outport  Tag=STV Outport  Port=203
  GaCDP_CellVolt_mV(95) : Outport  Tag=STV Outport  Port=204
  GaCDP_CellVolt_mV(96) : Outport  Tag=STV Outport  Port=205
  GaCDP_CellVolt_mV(97) : Outport  Tag=STV Outport  Port=206
  GaCDP_CellVolt_mV(98) : Outport  Tag=STV Outport  Port=207
  GaCDP_CellVolt_mV(99) : Outport  Tag=STV Outport  Port=208
  GaCDP_CellVolt_mV(100) : Outport  Tag=STV Outport  Port=209
  GaCDP_CellVolt_mV(101) : Outport  Tag=STV Outport  Port=210
  GaCDP_CellVolt_mV(102) : Outport  Tag=STV Outport  Port=211
  GaCDP_CellVolt_mV(103) : Outport  Tag=STV Outport  Port=212
  GaCDP_CellVolt_mV(104) : Outport  Tag=STV Outport  Port=213
  GaCDP_CellVolt_mV(105) : Outport  Tag=STV Outport  Port=214
  GaCDP_CellVolt_mV(106) : Outport  Tag=STV Outport  Port=215
  GaCDP_CellVolt_mV(107) : Outport  Tag=STV Outport  Port=216
  GaCDP_CellVolt_mV(108) : Outport  Tag=STV Outport  Port=217
  GaCDP_CellVolt_mV(109) : Outport  Tag=STV Outport  Port=218
  GaCDP_CellVolt_mV(110) : Outport  Tag=STV Outport  Port=219
  GaCDP_CellVolt_mV(111) : Outport  Tag=STV Outport  Port=220
  GaCDP_CellVolt_mV(112) : Outport  Tag=STV Outport  Port=221
  GeUDS_CapSel_enum : Outport  Tag=STV Outport  Port=222
  GbNVM_ReadLastShortSOCRunTiVld_flg : Outport  Tag=STV Outport  Port=223
  GcCDP_AvgCellVolt_mV : Outport  Tag=STV Outport  Port=224
  GcUDS_CellVoltNum_numb : Outport  Tag=STV Outport  Port=225
  GcHDP_PackCrnt_A : Outport  Tag=STV Outport  Port=226
  GeISP_WkUpSrcSt_enum : Outport  Tag=STV Outport  Port=227
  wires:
  FromWs/1 -> Demux/1
  Demux/1 -> GcCDP_MaxCellTemp_C/1
  Demux/2 -> GaCDP_CellTemp_C(1)/1
  Demux/3 -> GaCDP_CellTemp_C(2)/1
  Demux/4 -> GaCDP_CellTemp_C(3)/1
  Demux/5 -> GaCDP_CellTemp_C(4)/1
  Demux/6 -> GaCDP_CellTemp_C(5)/1
  Demux/7 -> GaCDP_CellTemp_C(6)/1
  Demux/8 -> GaCDP_CellTemp_C(7)/1
  Demux/9 -> GaCDP_CellTemp_C(8)/1
  Demux/10 -> GaCDP_CellTemp_C(9)/1
  Demux/11 -> GaCDP_CellTemp_C(10)/1
  Demux/12 -> GaCDP_CellTemp_C(11)/1
  Demux/13 -> GaCDP_CellTemp_C(12)/1
  Demux/14 -> GaCDP_CellTemp_C(13)/1
  Demux/15 -> GaCDP_CellTemp_C(14)/1
  Demux/16 -> GaCDP_CellTemp_C(15)/1
  Demux/17 -> GaCDP_CellTemp_C(16)/1
  Demux/18 -> GaCDP_CellTemp_C(17)/1
  Demux/19 -> GaCDP_CellTemp_C(18)/1
  Demux/20 -> GaCDP_CellTemp_C(19)/1
  Demux/21 -> GaCDP_CellTemp_C(20)/1
  Demux/22 -> GaCDP_CellTemp_C(21)/1
  Demux/23 -> GaCDP_CellTemp_C(22)/1
  Demux/24 -> GaCDP_CellTemp_C(23)/1
  Demux/25 -> GaCDP_CellTemp_C(24)/1
  Demux/26 -> GaCDP_CellTemp_C(25)/1
  Demux/27 -> GaCDP_CellTemp_C(26)/1
  Demux/28 -> GaCDP_CellTemp_C(27)/1
  Demux/29 -> GaCDP_CellTemp_C(28)/1
  Demux/30 -> GaCDP_CellTemp_C(29)/1
  Demux/31 -> GaCDP_CellTemp_C(30)/1
  Demux/32 -> GaCDP_CellTemp_C(31)/1
  Demux/33 -> GaCDP_CellTemp_C(32)/1
  Demux/34 -> GaCDP_CellTemp_C(33)/1
  Demux/35 -> GaCDP_CellTemp_C(34)/1
  Demux/36 -> GaCDP_CellTemp_C(35)/1
  Demux/37 -> GaCDP_CellTemp_C(36)/1
  Demux/38 -> GaCDP_CellTemp_C(37)/1
  Demux/39 -> GaCDP_CellTemp_C(38)/1
  Demux/40 -> GaCDP_CellTemp_C(39)/1
  Demux/41 -> GaCDP_CellTemp_C(40)/1
  Demux/42 -> GaCDP_CellTemp_C(41)/1
  Demux/43 -> GaCDP_CellTemp_C(42)/1
  Demux/44 -> GaCDP_CellTemp_C(43)/1
  Demux/45 -> GaCDP_CellTemp_C(44)/1
  Demux/46 -> GaCDP_CellTemp_C(45)/1
  Demux/47 -> GaCDP_CellTemp_C(46)/1
  Demux/48 -> GaCDP_CellTemp_C(47)/1
  Demux/49 -> GaCDP_CellTemp_C(48)/1
  Demux/50 -> GcCDP_MinCellTemp_C/1
  Demux/51 -> GcUDS_CellTempNumb_numb/1
  Demux/52 -> GcCDP_MaxBusbarTemp_C/1
  Demux/53 -> GcCDP_MinBusbarTemp_C/1
  Demux/54 -> GaCDP_BusbarTemp_C(1)/1
  Demux/55 -> GaCDP_BusbarTemp_C(2)/1
  Demux/56 -> GaCDP_BusbarTemp_C(3)/1
  Demux/57 -> GaCDP_BusbarTemp_C(4)/1
  Demux/58 -> GaCDP_BusbarTemp_C(5)/1
  Demux/59 -> GaCDP_BusbarTemp_C(6)/1
  Demux/60 -> GaCDP_BusbarTemp_C(7)/1
  Demux/61 -> GaCDP_BusbarTemp_C(8)/1
  Demux/62 -> GaCDP_BusbarTemp_C(9)/1
  Demux/63 -> GaCDP_BusbarTemp_C(10)/1
  Demux/64 -> GaCDP_BusbarTemp_C(11)/1
  Demux/65 -> GaCDP_BusbarTemp_C(12)/1
  Demux/66 -> GaCDP_BusbarTemp_C(13)/1
  Demux/67 -> GaCDP_BusbarTemp_C(14)/1
  Demux/68 -> GaCDP_BusbarTemp_C(15)/1
  Demux/69 -> GaCDP_BusbarTemp_C(16)/1
  Demux/70 -> GaCDP_BusbarTemp_C(17)/1
  Demux/71 -> GaCDP_BusbarTemp_C(18)/1
  Demux/72 -> GaCDP_BusbarTemp_C(19)/1
  Demux/73 -> GaCDP_BusbarTemp_C(20)/1
  Demux/74 -> GaCDP_BusbarTemp_C(21)/1
  Demux/75 -> GaCDP_BusbarTemp_C(22)/1
  Demux/76 -> GaCDP_BusbarTemp_C(23)/1
  Demux/77 -> GaCDP_BusbarTemp_C(24)/1
  Demux/78 -> GaCDP_BusbarTemp_C(25)/1
  Demux/79 -> GaCDP_BusbarTemp_C(26)/1
  Demux/80 -> GaCDP_BusbarTemp_C(27)/1
  Demux/81 -> GaCDP_BusbarTemp_C(28)/1
  Demux/82 -> GaCDP_BusbarTemp_C(29)/1
  Demux/83 -> GaCDP_BusbarTemp_C(30)/1
  Demux/84 -> GaCDP_BusbarTemp_C(31)/1
  Demux/85 -> GaCDP_BusbarTemp_C(32)/1
  Demux/86 -> GaCDP_BusbarTemp_C(33)/1
  Demux/87 -> GaCDP_BusbarTemp_C(34)/1
  Demux/88 -> GaCDP_BusbarTemp_C(35)/1
  Demux/89 -> GaCDP_BusbarTemp_C(36)/1
  Demux/90 -> GaCDP_BusbarTemp_C(37)/1
  Demux/91 -> GaCDP_BusbarTemp_C(38)/1
  Demux/92 -> GaCDP_BusbarTemp_C(39)/1
  Demux/93 -> GaCDP_BusbarTemp_C(40)/1
  Demux/94 -> GaCDP_BusbarTemp_C(41)/1
  Demux/95 -> GaCDP_BusbarTemp_C(42)/1
  Demux/96 -> GaCDP_BusbarTemp_C(43)/1
  Demux/97 -> GaCDP_BusbarTemp_C(44)/1
  Demux/98 -> GaCDP_BusbarTemp_C(45)/1
  Demux/99 -> GaCDP_BusbarTemp_C(46)/1
  Demux/100 -> GaCDP_BusbarTemp_C(47)/1
  Demux/101 -> GaCDP_BusbarTemp_C(48)/1
  Demux/102 -> GcUDS_BusbarTempNumb_numb/1
  Demux/103 -> GeMSM_BMUState_enum/1
  Demux/104 -> GbCDP_SumCellVoltVld_flg/1
  Demux/105 -> GcRTC_SleepTime_min/1
  Demux/106 -> GbNVM_ReadShortSOCIDFitVld_flg/1
  Demux/107 -> GbNVM_ReadShortSOCMinIDVld_flg/1
  Demux/108 -> GbNVM_ReadShortSOCDiffVld_flg/1
  Demux/109 -> GbNVM_ReadShortSOCRunTiSumVld_flg/1
  Demux/110 -> GaCDP_CellVolt_mV(1)/1
  Demux/111 -> GaCDP_CellVolt_mV(2)/1
  Demux/112 -> GaCDP_CellVolt_mV(3)/1
  Demux/113 -> GaCDP_CellVolt_mV(4)/1
  Demux/114 -> GaCDP_CellVolt_mV(5)/1
  Demux/115 -> GaCDP_CellVolt_mV(6)/1
  Demux/116 -> GaCDP_CellVolt_mV(7)/1
  Demux/117 -> GaCDP_CellVolt_mV(8)/1
  Demux/118 -> GaCDP_CellVolt_mV(9)/1
  Demux/119 -> GaCDP_CellVolt_mV(10)/1
  Demux/120 -> GaCDP_CellVolt_mV(11)/1
  Demux/121 -> GaCDP_CellVolt_mV(12)/1
  Demux/122 -> GaCDP_CellVolt_mV(13)/1
  Demux/123 -> GaCDP_CellVolt_mV(14)/1
  Demux/124 -> GaCDP_CellVolt_mV(15)/1
  Demux/125 -> GaCDP_CellVolt_mV(16)/1
  Demux/126 -> GaCDP_CellVolt_mV(17)/1
  Demux/127 -> GaCDP_CellVolt_mV(18)/1
  Demux/128 -> GaCDP_CellVolt_mV(19)/1
  Demux/129 -> GaCDP_CellVolt_mV(20)/1
  Demux/130 -> GaCDP_CellVolt_mV(21)/1
  Demux/131 -> GaCDP_CellVolt_mV(22)/1
  Demux/132 -> GaCDP_CellVolt_mV(23)/1
  Demux/133 -> GaCDP_CellVolt_mV(24)/1
  Demux/134 -> GaCDP_CellVolt_mV(25)/1
  Demux/135 -> GaCDP_CellVolt_mV(26)/1
  Demux/136 -> GaCDP_CellVolt_mV(27)/1
  Demux/137 -> GaCDP_CellVolt_mV(28)/1
  Demux/138 -> GaCDP_CellVolt_mV(29)/1
  Demux/139 -> GaCDP_CellVolt_mV(30)/1
  Demux/140 -> GaCDP_CellVolt_mV(31)/1
  Demux/141 -> GaCDP_CellVolt_mV(32)/1
  Demux/142 -> GaCDP_CellVolt_mV(33)/1
  Demux/143 -> GaCDP_CellVolt_mV(34)/1
  Demux/144 -> GaCDP_CellVolt_mV(35)/1
  Demux/145 -> GaCDP_CellVolt_mV(36)/1
  Demux/146 -> GaCDP_CellVolt_mV(37)/1
  Demux/147 -> GaCDP_CellVolt_mV(38)/1
  Demux/148 -> GaCDP_CellVolt_mV(39)/1
  Demux/149 -> GaCDP_CellVolt_mV(40)/1
  Demux/150 -> GaCDP_CellVolt_mV(41)/1
  Demux/151 -> GaCDP_CellVolt_mV(42)/1
  Demux/152 -> GaCDP_CellVolt_mV(43)/1
  Demux/153 -> GaCDP_CellVolt_mV(44)/1
  Demux/154 -> GaCDP_CellVolt_mV(45)/1
  Demux/155 -> GaCDP_CellVolt_mV(46)/1
  Demux/156 -> GaCDP_CellVolt_mV(47)/1
  Demux/157 -> GaCDP_CellVolt_mV(48)/1
  Demux/158 -> GaCDP_CellVolt_mV(49)/1
  Demux/159 -> GaCDP_CellVolt_mV(50)/1
  Demux/160 -> GaCDP_CellVolt_mV(51)/1
  Demux/161 -> GaCDP_CellVolt_mV(52)/1
  Demux/162 -> GaCDP_CellVolt_mV(53)/1
  Demux/163 -> GaCDP_CellVolt_mV(54)/1
  Demux/164 -> GaCDP_CellVolt_mV(55)/1
  Demux/165 -> GaCDP_CellVolt_mV(56)/1
  Demux/166 -> GaCDP_CellVolt_mV(57)/1
  Demux/167 -> GaCDP_CellVolt_mV(58)/1
  Demux/168 -> GaCDP_CellVolt_mV(59)/1
  Demux/169 -> GaCDP_CellVolt_mV(60)/1
  Demux/170 -> GaCDP_CellVolt_mV(61)/1
  Demux/171 -> GaCDP_CellVolt_mV(62)/1
  Demux/172 -> GaCDP_CellVolt_mV(63)/1
  Demux/173 -> GaCDP_CellVolt_mV(64)/1
  Demux/174 -> GaCDP_CellVolt_mV(65)/1
  Demux/175 -> GaCDP_CellVolt_mV(66)/1
  Demux/176 -> GaCDP_CellVolt_mV(67)/1
  Demux/177 -> GaCDP_CellVolt_mV(68)/1
  Demux/178 -> GaCDP_CellVolt_mV(69)/1
  Demux/179 -> GaCDP_CellVolt_mV(70)/1
  Demux/180 -> GaCDP_CellVolt_mV(71)/1
  Demux/181 -> GaCDP_CellVolt_mV(72)/1
  Demux/182 -> GaCDP_CellVolt_mV(73)/1
  Demux/183 -> GaCDP_CellVolt_mV(74)/1
  Demux/184 -> GaCDP_CellVolt_mV(75)/1
  Demux/185 -> GaCDP_CellVolt_mV(76)/1
  Demux/186 -> GaCDP_CellVolt_mV(77)/1
  Demux/187 -> GaCDP_CellVolt_mV(78)/1
  Demux/188 -> GaCDP_CellVolt_mV(79)/1
  Demux/189 -> GaCDP_CellVolt_mV(80)/1
  Demux/190 -> GaCDP_CellVolt_mV(81)/1
  Demux/191 -> GaCDP_CellVolt_mV(82)/1
  Demux/192 -> GaCDP_CellVolt_mV(83)/1
  Demux/193 -> GaCDP_CellVolt_mV(84)/1
  Demux/194 -> GaCDP_CellVolt_mV(85)/1
  Demux/195 -> GaCDP_CellVolt_mV(86)/1
  Demux/196 -> GaCDP_CellVolt_mV(87)/1
  Demux/197 -> GaCDP_CellVolt_mV(88)/1
  Demux/198 -> GaCDP_CellVolt_mV(89)/1
  Demux/199 -> GaCDP_CellVolt_mV(90)/1
  Demux/200 -> GaCDP_CellVolt_mV(91)/1
  Demux/201 -> GaCDP_CellVolt_mV(92)/1
  Demux/202 -> GaCDP_CellVolt_mV(93)/1
  Demux/203 -> GaCDP_CellVolt_mV(94)/1
  Demux/204 -> GaCDP_CellVolt_mV(95)/1
  Demux/205 -> GaCDP_CellVolt_mV(96)/1
  Demux/206 -> GaCDP_CellVolt_mV(97)/1
  Demux/207 -> GaCDP_CellVolt_mV(98)/1
  Demux/208 -> GaCDP_CellVolt_mV(99)/1
  Demux/209 -> GaCDP_CellVolt_mV(100)/1
  Demux/210 -> GaCDP_CellVolt_mV(101)/1
  Demux/211 -> GaCDP_CellVolt_mV(102)/1
  Demux/212 -> GaCDP_CellVolt_mV(103)/1
  Demux/213 -> GaCDP_CellVolt_mV(104)/1
  Demux/214 -> GaCDP_CellVolt_mV(105)/1
  Demux/215 -> GaCDP_CellVolt_mV(106)/1
  Demux/216 -> GaCDP_CellVolt_mV(107)/1
  Demux/217 -> GaCDP_CellVolt_mV(108)/1
  Demux/218 -> GaCDP_CellVolt_mV(109)/1
  Demux/219 -> GaCDP_CellVolt_mV(110)/1
  Demux/220 -> GaCDP_CellVolt_mV(111)/1
  Demux/221 -> GaCDP_CellVolt_mV(112)/1
  Demux/222 -> GeUDS_CapSel_enum/1
  Demux/223 -> GbNVM_ReadLastShortSOCRunTiVld_flg/1
  Demux/224 -> GcCDP_AvgCellVolt_mV/1
  Demux/225 -> GcUDS_CellVoltNum_numb/1
  Demux/226 -> GcHDP_PackCrnt_A/1
  Demux/227 -> GeISP_WkUpSrcSt_enum/1
